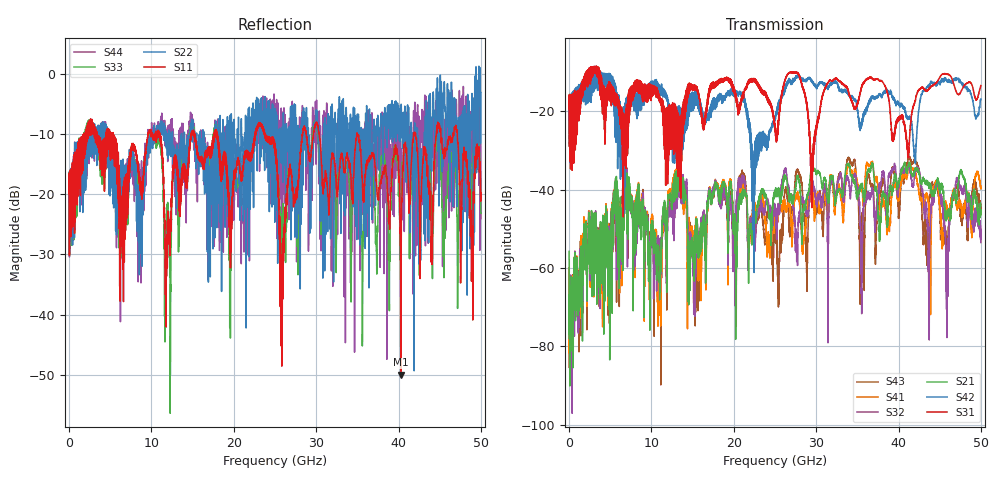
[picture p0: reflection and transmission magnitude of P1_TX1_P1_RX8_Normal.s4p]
!Keysight Technologies,N5225B,MY57041031,A.13.20.10
!Date: Friday, May 31, 2019 11:25:35
!Correction: S11(Full 4 Port(1,2,3,4))
!S12(Full 4 Port(1,2,3,4))
!S13(Full 4 Port(1,2,3,4))
!S14(Full 4 Port(1,2,3,4))
!S21(Full 4 Port(1,2,3,4))
!S22(Full 4 Port(1,2,3,4))
!S23(Full 4 Port(1,2,3,4))
!S24(Full 4 Port(1,2,3,4))
!S31(Full 4 Port(1,2,3,4))
!S32(Full 4 Port(1,2,3,4))
!S33(Full 4 Port(1,2,3,4))
!S34(Full 4 Port(1,2,3,4))
!S41(Full 4 Port(1,2,3,4))
!S42(Full 4 Port(1,2,3,4))
!S43(Full 4 Port(1,2,3,4))
!S44(Full 4 Port(1,2,3,4))
!S4P File: Measurements: <S11,S12,S13,S14>,
!<S21,S22,S23,S24>,
!<S31,S32,S33,S34>,
!<S41,S42,S43,S44>:
# Hz S  dB  R 50.0
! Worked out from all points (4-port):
!   5000 points, 10 MHz to 50 GHz, reference 50 ohm
!   strongest paths, dB at 10 MHz, 12.51 GHz, 25.01 GHz, 37.51 GHz, 50 GHz:
!     S31: -19.3, -29.3, -24.5, -11.8, -13.4
!     S42: -19.4, -24.4, -22.3, -16.3, -16.9
!     S21: -55.8, -42.9, -41.4, -45.1, -46.5
!     S32: -69.7, -43.5, -46.2, -41.6, -53.5
!     S41: -64.9, -40.7, -48.4, -39.3, -39.6
!     S43: -60.0, -41.3, -52.6, -44.6, -44.8
!   lowest |S11| = -50.0 dB at 40.27 GHz (marker M1), VSWR 1.01, Z = 49.7 + j0.0787 ohm
!   |S11| at or under -10 dB: 18.01 GHz to 22.61 GHz (4.596 GHz wide, 22.6 % of centre); 30.38 GHz to 34.94 GHz (4.561 GHz wide, 14 % of centre); 34.98 GHz to 41.81 GHz (6.837 GHz wide, 17.8 % of centre)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
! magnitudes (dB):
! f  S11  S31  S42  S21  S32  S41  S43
! 10 MHz  -19.9  -19.3  -19.4  -55.8  -69.7  -64.9  -60.0
! 5.65 GHz  -11.5  -16.8  -19.0  -37.2  -38.3  -37.5  -38.8
! 10.93 GHz  -10.2  -16.5  -13.6  -58.5  -54.3  -58.1  -57.3
! 13.09 GHz  -15.6  -22.7  -19.3  -35.8  -36.6  -35.5  -36.1
! 25.46 GHz  -21.8  -21.2  -18.7  -40.8  -45.6  -45.4  -64.7
! 40.27 GHz  -50.0  -21.3  -18.1  -36.2  -35.5  -38.4  -39.6
! 50 GHz  -19.7  -13.4  -16.9  -46.5  -53.5  -39.6  -44.8
